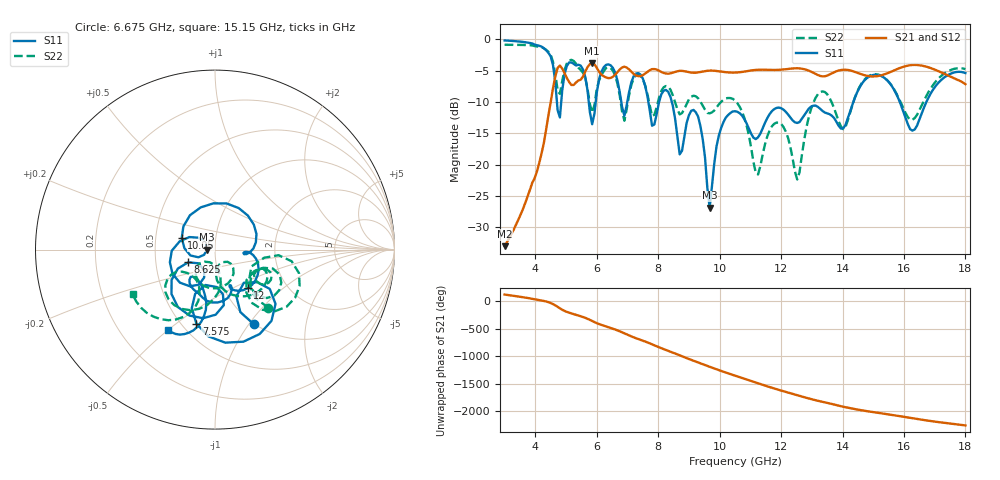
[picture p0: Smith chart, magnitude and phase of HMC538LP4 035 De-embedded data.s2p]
! Chelmsford, MA 01824
! http://www.hittite.com
! Tel: 978-250-3343
! Fax: 978-250-3373
! Device  :  HMC538LP4
! Description:  600 Analog Phase Shifter
! Frequency  :  6.0 GHz - 15.0 GHz
! Package  :  LP4  - 4x4 mm Quad Flatpack No-Lead (QFN) Plastic Package: 24 pin
! Ports  :  2 RF, 1 DC
!  Pin  3  = Rfin  = Port 1
!  Pin  16  = Rfout = Port 2
!  pin  21  = vCTL
! Voltages:  VCTL  = 0 to 5.0 Volts
! Currents :  Vb(V)  Vd(V)  Ib(mA)  Id(mA)
!  0.00  3.50  0.000000	0.479475
! Data:  The device was measured on evaluation board 111296-1.
!  Data was collected using a calibrated network analyzer.
!  The evaluation circuit board was modeled and simulated.This was use
!  to removed the evaluation board circuit from the measured data.
!  The reference plane is the center of the package pin.
! Misc:  Lot #
!Date Measured:  03 - 11 -2009
! Date:  03 - 17 -2009
! Note:
!  Hittite Microwave supplies this data as a sample of measured data at the
!  package pin for this package product.  Your particular data for this product
!  may vary.
!  Data was taken at 25 degrees C.
!  Hittite Microwave reserves the right to change this data at anytime.
# MHz S MA R 50
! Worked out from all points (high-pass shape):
!   201 points, 3 GHz to 18 GHz, reference 50 ohm
!   highest |S21| = -3.85 dB at 5.85 GHz (marker M1); lowest = -33.0 dB at 3 GHz (marker M2)
!   |S21| within 3 dB of the highest: 4.614 GHz to 5.103 GHz (489.1 MHz wide, 10.1 % of centre); 5.34 GHz to 17.9 GHz (12.56 GHz wide, 108 % of centre)
!   lowest |S11| = -26.9 dB at 9.675 GHz (marker M3), VSWR 1.09, Z = 45.7 + j0.0271 ohm
!   |S11| at or under -10 dB: 7.68 GHz to 8.03 GHz (349.9 MHz wide, 4.45 % of centre); 8.443 GHz to 14.35 GHz (5.911 GHz wide, 51.9 % of centre); 15.86 GHz to 16.73 GHz (868.9 MHz wide, 5.33 % of centre)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
!   |S22| runs from -22.4 to -0.9 dB; largest |S21 - S12| = 0.003
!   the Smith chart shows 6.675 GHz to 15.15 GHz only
!   S11 on the Smith chart (normalised r, x): 6.675 GHz: 0.99, -1.05; 7.575 GHz: 0.59, -0.59; 8.625 GHz: 0.73, -0.11; 10.05 GHz: 0.68, +0.09; 12 GHz: 1.29, -0.60; 15.15 GHz: 0.41, -0.50
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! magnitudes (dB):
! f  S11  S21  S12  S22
! 3 GHz  -0.2  -33.0  -33.0  -0.9
! 4.425 GHz  -2.2  -12.2  -12.2  -2.0
! 4.725 GHz  -11.3  -4.6  -4.6  -8.1
! 5.55 GHz  -4.8  -6.0  -6.0  -5.4
! 5.85 GHz  -13.6  -3.8  -3.9  -11.7
! 6.675 GHz  -6.6  -5.2  -5.2  -7.1
! 7.575 GHz  -7.4  -5.5  -5.5  -7.4
! 8.025 GHz  -10.1  -5.0  -5.0  -9.4
! 8.625 GHz  -15.6  -5.1  -5.1  -11.2
! 9.3 GHz  -12.4  -5.3  -5.3  -9.4
! 9.675 GHz  -26.9  -5.0  -5.0  -11.8
! 10.05 GHz  -14.1  -5.2  -5.2  -10.0
! 10.5 GHz  -11.5  -5.3  -5.3  -9.8
! 11.25 GHz  -15.7  -4.9  -4.9  -21.6
! 12 GHz  -11.0  -4.9  -4.9  -13.5
! 12.53 GHz  -13.4  -4.6  -4.7  -22.4
! 13.05 GHz  -10.6  -5.4  -5.4  -10.1
! 14.03 GHz  -14.2  -4.9  -4.9  -14.4
! 15.15 GHz  -5.7  -5.9  -5.9  -5.6
! 15.53 GHz  -6.9  -5.3  -5.3  -6.9
! 16.27 GHz  -14.6  -4.1  -4.1  -12.9
! 18 GHz  -5.4  -7.2  -7.2  -4.8
